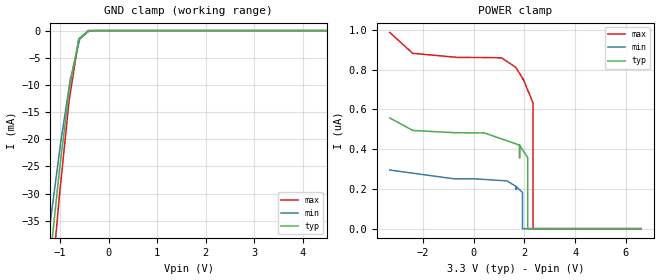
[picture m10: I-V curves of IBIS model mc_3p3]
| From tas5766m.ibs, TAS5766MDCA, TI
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|   mc_3p3 Model
[Model]   mc_3p3
Model_type   Input
Vinl = 0.99
Vinh = 2.31
|   typ   min   max
C_comp   0.996pF   0.979pF   1.002pF
[Voltage Range]   3.3   3   3.6
[Temperature Range]   27   105   -25
[Power Clamp Reference]   3.3   3   3.6
[GND Clamp Reference]   -0   -0   -0
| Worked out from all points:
|   GND clamp passes 1 mA (typ) near -0.54 V on its own axis
[GND Clamp]
|   Voltage   I(typ)   I(min)   I(max)
-3.3V     -526.2mA   -489.4mA   -552.7mA
-1.384V   -58.51mA   -49.12mA   -68.56mA
-1.208V   -42.45mA   -36.01mA   -49.95mA
-1.186V   -40.51mA   -34.34mA   -47.72mA
-1.01V    -25.63mA   -22.28mA   -30.25mA
-806.5mV  -10.7mA    -10.07mA   -12.62mA
-789.9mV  -9.929mA   -9.096mA   -11.67mA
-614.3mV  -1.741mA   -2.396mA   -1.619mA
-591.9mV  -1.35mA    -1.541mA   -1.436mA
-416.3mV  -55.48uA   -203.6uA   -6.973uA
-195.9mV  -8.44uA    -191.8nA   -120.7nA
6.6V      0A         0A         0A
[POWER Clamp]
|   Voltage   I(typ)   I(min)   I(max)
-3.3V     557nA      295.1nA    987.6nA
1.664V    426.9nA    213.3nA    811.6nA
1.926V    398nA      182.2nA    757.5nA
1.927V    397.7nA    0A         757.2nA
2.133V    356.8nA    0A         697.4nA
2.133V    323.7nA    0A         697.3nA
2.134V    0A         0A         697.2nA
2.341V    0A         0A         631.6nA
2.342V    0A         0A         593.6nA
2.342V    0A         0A         422.9nA
2.342V    0A         0A         0A
6.6V      0A         0A         0A
